FUNCTION_BLOCK Example06_sync //4x3 flyways, 4 xbots - get xbot prop, set xbot prop, sync move
VAR_INPUT
	Execute : BOOL;
END_VAR
VAR_OUTPUT
	Done : BOOL;
END_VAR
VAR_IN_OUT
	PM_Controller : PMControllerType;	// the planar motor controller to use
END_VAR
VAR
	xbotID_array78 : ARRAY[0..77] OF USINT;
	PosX_array78 : ARRAY[0..77] OF REAL;
	PosY_array78 : ARRAY[0..77] OF REAL;
	PMC_AutoDrivingMotion1 : PMC_AutoDrivingMotion;
	xbotID_array14 : ARRAY[0..13] OF USINT;
	xbotprop_array14 : ARRAY[0..13] OF USINT;
	propvalue_array14 : ARRAY[0..13] OF REAL;
	PMC_SetXbotProperty1 : PMC_SetXbotProperty;
	payload1 : REAL;
	PMC_GetXbotProperty1 : PMC_GetXbotProperty;
	xbotID_array4 : ARRAY[0..3] OF USINT;
	endvel_4 : ARRAY[0..3] OF REAL;
	posx_4 : ARRAY[0..3] OF REAL;
	posy_4 : ARRAY[0..3] OF REAL;
	maxacc_4 : ARRAY[0..3] OF REAL;
	maxvel_4 : ARRAY[0..3] OF REAL;
	PMC_SyncMotion1 : PMC_SyncMotion;
	PMC_SetXbotProperty2 : PMC_SetXbotProperty;
	payload2 : REAL;
	PMC_GetXbotProperty2 : PMC_GetXbotProperty;
	PMC_SyncMotion2 : PMC_SyncMotion;
END_VAR

//4x3 flyways, 4 xbots - get xbot prop, set xbot prop, sync move

//async move to 60,60 300,60 540,60 780,60
xbotID_array78[0] := 1;xbotID_array78[1] := 2;xbotID_array78[2] := 3;xbotID_array78[3] := 4;
PosX_array78[0] := 0.060;PosX_array78[1] := 0.300;PosX_array78[2] := 0.540;PosX_array78[3] := 0.780;
PosY_array78[0] := 0.060;PosY_array78[1] := 0.060;PosY_array78[2] := 0.060;PosY_array78[3] := 0.060;
PMC_AutoDrivingMotion1(Execute := Execute,nXbots := 4,RoutingType := 0,ZoneID := 0,XbotID := xbotID_array78,PosX := PosX_array78,PosY := PosY_array78,PM_Controller := PM_Controller);

//set payload weight of all xbots to 0.55 kg
xbotID_array14[0] := 1;xbotID_array14[1] := 2;xbotID_array14[2] := 3;xbotID_array14[3] := 4;
xbotprop_array14[0] := 1;xbotprop_array14[1] := 1;xbotprop_array14[2] := 1;xbotprop_array14[3] := 1;
propvalue_array14[0] := 0.55;propvalue_array14[1] := 0.55;propvalue_array14[2] := 0.55;propvalue_array14[3] := 0.55;
PMC_SetXbotProperty1(Execute := PMC_AutoDrivingMotion1.Done,nXbots := 4,XbotID := xbotID_array14,PropertyID := xbotprop_array14,Value := propvalue_array14,PM_Controller := PM_Controller);

//read payload weight of xbot 2
PMC_GetXbotProperty1(Execute := PMC_SetXbotProperty1.Done,XbotID := 2,PayloadW => payload1,PM_Controller := PM_Controller);

//sync move all xbots to top of flyways
xbotID_array4[0] := 1;xbotID_array4[1] := 2;xbotID_array4[2] := 3;xbotID_array4[3] := 4;
endvel_4[0] := 0.0;endvel_4[1] := 0.0;endvel_4[2] := 0.0;endvel_4[3] := 0.0;
posx_4[0] := 0.06;posx_4[1] := 0.30;posx_4[2] := 0.54;posx_4[3] := 0.78;
posy_4[0] := 0.66;posy_4[1] := 0.66;posy_4[2] := 0.66;posy_4[3] := 0.66;
maxacc_4[0] := 20;maxacc_4[1] := 20;maxacc_4[2] := 20;maxacc_4[3] := 20;
maxvel_4[0] := 2;maxvel_4[1] := 2;maxvel_4[2] := 2;maxvel_4[3] := 2;
PMC_SyncMotion1(Execute := PMC_GetXbotProperty1.Valid,nXbots := 4,XbotID := xbotID_array4,PosX := posx_4,PosY := posy_4,EndVel := endvel_4,MaxVel := maxvel_4,MaxAcc := maxacc_4,PM_Controller := PM_Controller);

//set payload weight of all xbots to 0.0 kg
xbotID_array14[0] := 1;xbotID_array14[1] := 2;xbotID_array14[2] := 3;xbotID_array14[3] := 4;
xbotprop_array14[0] := 1;xbotprop_array14[1] := 1;xbotprop_array14[2] := 1;xbotprop_array14[3] := 1;
propvalue_array14[0] := 0.0;propvalue_array14[1] := 0.0;propvalue_array14[2] := 0.0;propvalue_array14[3] := 0.0;	
PMC_SetXbotProperty2(Execute := PMC_SyncMotion1.Done,nXbots := 4,XbotID := xbotID_array14,PropertyID := xbotprop_array14,Value := propvalue_array14,PM_Controller := PM_Controller);

//read payload weight of xbot 3
PMC_GetXbotProperty2(Execute := PMC_SetXbotProperty2.Done,XbotID := 3,PayloadW => payload2,PM_Controller := PM_Controller);

//sync move all xbots to bottom of flyways
xbotID_array4[0] := 1;xbotID_array4[1] := 2;xbotID_array4[2] := 3;xbotID_array4[3] := 4;
endvel_4[0] := 0.0;endvel_4[1] := 0.0;endvel_4[2] := 0.0;endvel_4[3] := 0.0;
posx_4[0] := 0.06;posx_4[1] := 0.30;posx_4[2] := 0.54;posx_4[3] := 0.78;
posy_4[0] := 0.06;posy_4[1] := 0.06;posy_4[2] := 0.06;posy_4[3] := 0.06;
maxacc_4[0] := 20;maxacc_4[1] := 20;maxacc_4[2] := 20;maxacc_4[3] := 20;
maxvel_4[0] := 2;maxvel_4[1] := 2;maxvel_4[2] := 2;maxvel_4[3] := 2;
PMC_SyncMotion2(Execute := PMC_GetXbotProperty2.Valid,nXbots := 4,XbotID := xbotID_array4,PosX := posx_4,PosY := posy_4,EndVel := endvel_4,MaxVel := maxvel_4,MaxAcc := maxacc_4,PM_Controller := PM_Controller);

Done := PMC_SyncMotion2.Done;

END_FUNCTION_BLOCK
